(* Logix 5000 AddOnInstructionDefinition export SPEL_Above; software revision 30.01; part 5 of 9 *)

ADD_ON_INSTRUCTION SPEL_LocalSet   (* revision 1.0, vendor SEIKO EPSON CORP. *)
// Sets the local coordinate system of the specified coordinate number by each coordinate.
VAR_INPUT
   Start : BOOL; {required}
END_VAR
VAR_OUTPUT
   InCycle : BOOL; {access Read Only, visible}
   Done : BOOL; {access Read Only, visible}
   Error : BOOL; {access Read Only, visible}
END_VAR
VAR_INPUT
   NumAxes : INT; {required}
   LocalNum : INT; {required}
   LocalX : REAL; {required}
   LocalY : REAL; {required}
   LocalZ : REAL; {required}
   LocalU : REAL; {required}
   LocalV : REAL; {required}
   LocalW : REAL; {required}
END_VAR
VAR_IN_OUT
   ExtInputs : AB:ETHERNET_MODULE_INT_128Bytes:I:0; {required}
   ExtOutputs : AB:ETHERNET_MODULE_INT_128Bytes:O:0; {required}
END_VAR
VAR_OUTPUT
   ErrCode1 : INT; {access Read Only, visible}
   ErrCode2 : INT; {access Read Only, visible}
END_VAR
VAR
   Coordinatex1000 : DINT; {access None}
   Coordinate_INTS : INT[2]; {access None}
   ExecLocalSetZ : SPEL_ExecCmd := (MaxTime := 3000); {access None}
   ExecLocalSetY : SPEL_ExecCmd := (MaxTime := 3000); {access None}
   ExecLocalSetX : SPEL_ExecCmd := (MaxTime := 3000); {access None}
   X6 : BOOL; {access None}
   StartInit : BOOL[32]; {access None}
   OneShotStart : BOOL[32]; {access None}
   ExecLocalSetW : SPEL_ExecCmd := (MaxTime := 3000); {access None}
   ExecLocalSetV : SPEL_ExecCmd := (MaxTime := 3000); {access None}
   ExecLocalSetU : SPEL_ExecCmd := (MaxTime := 3000); {access None}
   ExecTimeout : DINT; {access None}
END_VAR

ROUTINE Logic   (* ladder *)
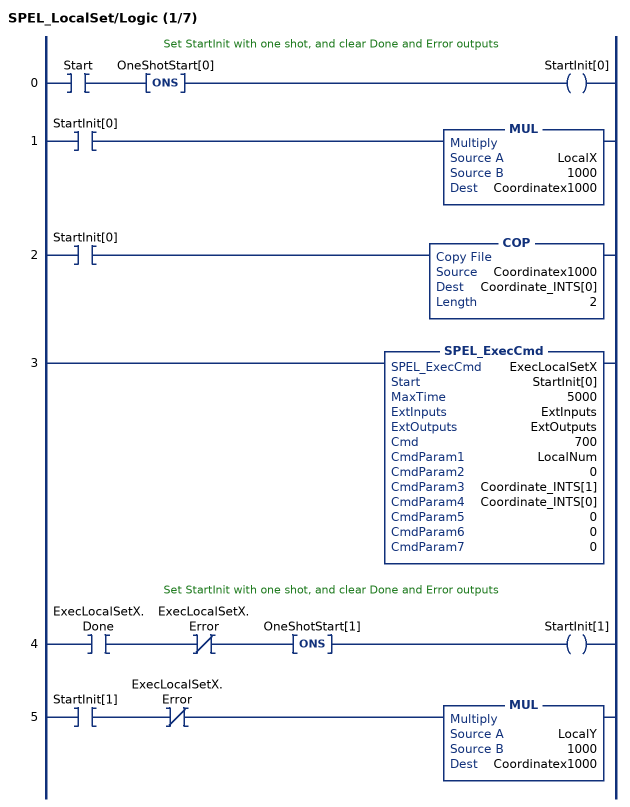
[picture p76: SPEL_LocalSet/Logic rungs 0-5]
   // Set StartInit with one shot, and clear Done and Error outputs
   0: XIC(Start)ONS(OneShotStart[0])OTE(StartInit[0]);
   1: XIC(StartInit[0])MUL(LocalX,1000,Coordinatex1000);
   2: XIC(StartInit[0])COP(Coordinatex1000,Coordinate_INTS[0],2);
   3: SPEL_ExecCmd(ExecLocalSetX,StartInit[0],5000,ExtInputs,ExtOutputs,700,LocalNum,0,Coordinate_INTS[1],Coordinate_INTS[0],0,0,0);
   // Set StartInit with one shot, and clear Done and Error outputs
   4: XIC(ExecLocalSetX.Done)XIO(ExecLocalSetX.Error)ONS(OneShotStart[1])OTE(StartInit[1]);
   5: XIC(StartInit[1])XIO(ExecLocalSetX.Error)MUL(LocalY,1000,Coordinatex1000);
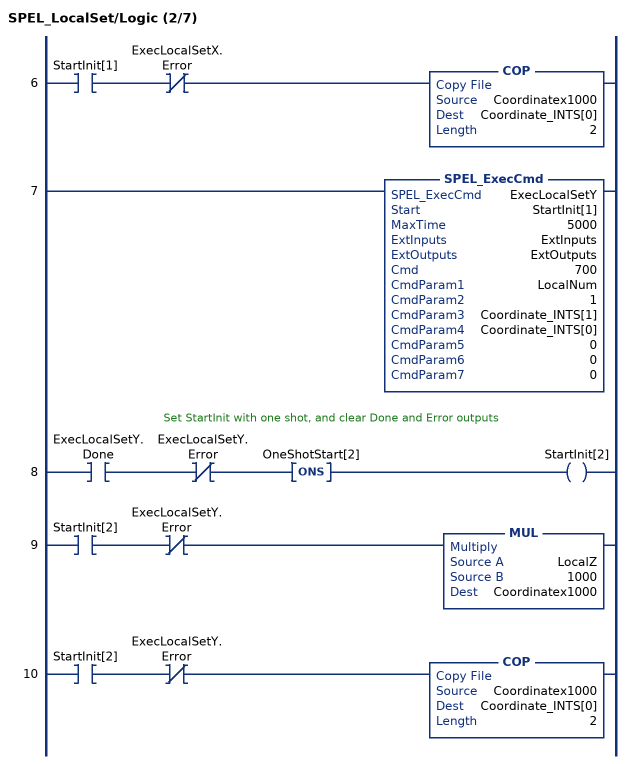
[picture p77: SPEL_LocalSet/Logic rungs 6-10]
   6: XIC(StartInit[1])XIO(ExecLocalSetX.Error)COP(Coordinatex1000,Coordinate_INTS[0],2);
   7: SPEL_ExecCmd(ExecLocalSetY,StartInit[1],5000,ExtInputs,ExtOutputs,700,LocalNum,1,Coordinate_INTS[1],Coordinate_INTS[0],0,0,0);
   // Set StartInit with one shot, and clear Done and Error outputs
   8: XIC(ExecLocalSetY.Done)XIO(ExecLocalSetY.Error)ONS(OneShotStart[2])OTE(StartInit[2]);
   9: XIC(StartInit[2])XIO(ExecLocalSetY.Error)MUL(LocalZ,1000,Coordinatex1000);
   10: XIC(StartInit[2])XIO(ExecLocalSetY.Error)COP(Coordinatex1000,Coordinate_INTS[0],2);
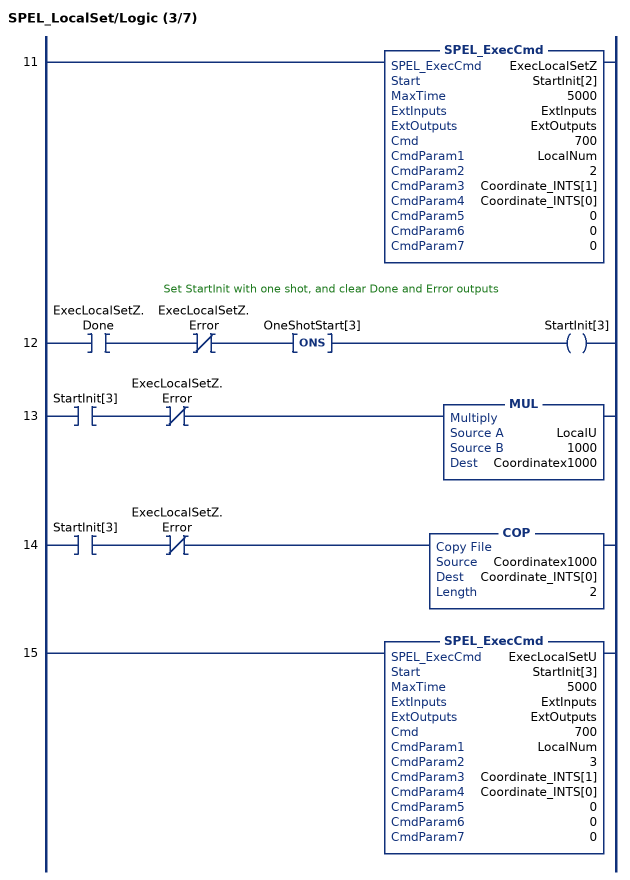
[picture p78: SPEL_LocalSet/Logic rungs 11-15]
   11: SPEL_ExecCmd(ExecLocalSetZ,StartInit[2],5000,ExtInputs,ExtOutputs,700,LocalNum,2,Coordinate_INTS[1],Coordinate_INTS[0],0,0,0);
   // Set StartInit with one shot, and clear Done and Error outputs
   12: XIC(ExecLocalSetZ.Done)XIO(ExecLocalSetZ.Error)ONS(OneShotStart[3])OTE(StartInit[3]);
   13: XIC(StartInit[3])XIO(ExecLocalSetZ.Error)MUL(LocalU,1000,Coordinatex1000);
   14: XIC(StartInit[3])XIO(ExecLocalSetZ.Error)COP(Coordinatex1000,Coordinate_INTS[0],2);
   15: SPEL_ExecCmd(ExecLocalSetU,StartInit[3],5000,ExtInputs,ExtOutputs,700,LocalNum,3,Coordinate_INTS[1],Coordinate_INTS[0],0,0,0);
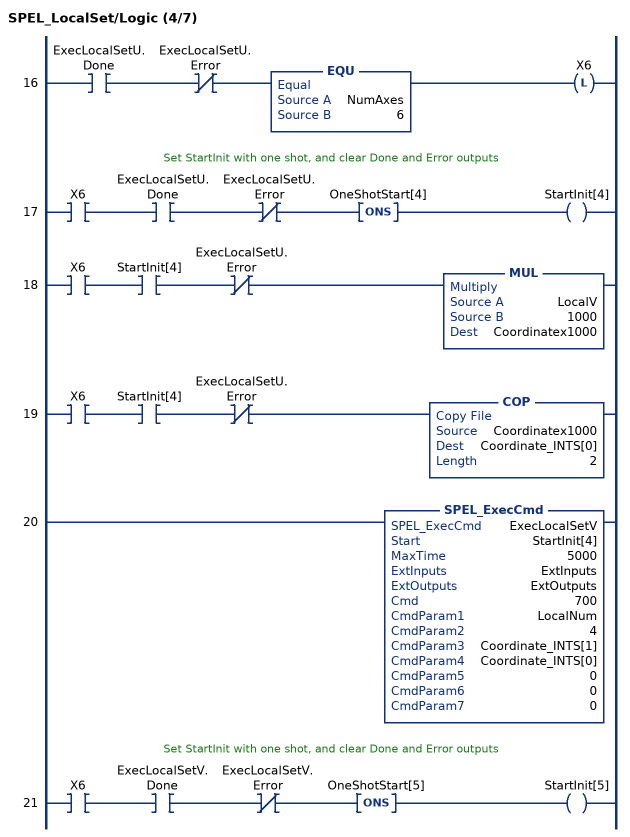
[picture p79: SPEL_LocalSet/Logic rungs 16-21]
   16: XIC(ExecLocalSetU.Done)XIO(ExecLocalSetU.Error)EQU(NumAxes,6)OTL(X6);
   // Set StartInit with one shot, and clear Done and Error outputs
   17: XIC(X6)XIC(ExecLocalSetU.Done)XIO(ExecLocalSetU.Error)ONS(OneShotStart[4])OTE(StartInit[4]);
   18: XIC(X6)XIC(StartInit[4])XIO(ExecLocalSetU.Error)MUL(LocalV,1000,Coordinatex1000);
   19: XIC(X6)XIC(StartInit[4])XIO(ExecLocalSetU.Error)COP(Coordinatex1000,Coordinate_INTS[0],2);
   20: SPEL_ExecCmd(ExecLocalSetV,StartInit[4],5000,ExtInputs,ExtOutputs,700,LocalNum,4,Coordinate_INTS[1],Coordinate_INTS[0],0,0,0);
   // Set StartInit with one shot, and clear Done and Error outputs
   21: XIC(X6)XIC(ExecLocalSetV.Done)XIO(ExecLocalSetV.Error)ONS(OneShotStart[5])OTE(StartInit[5]);
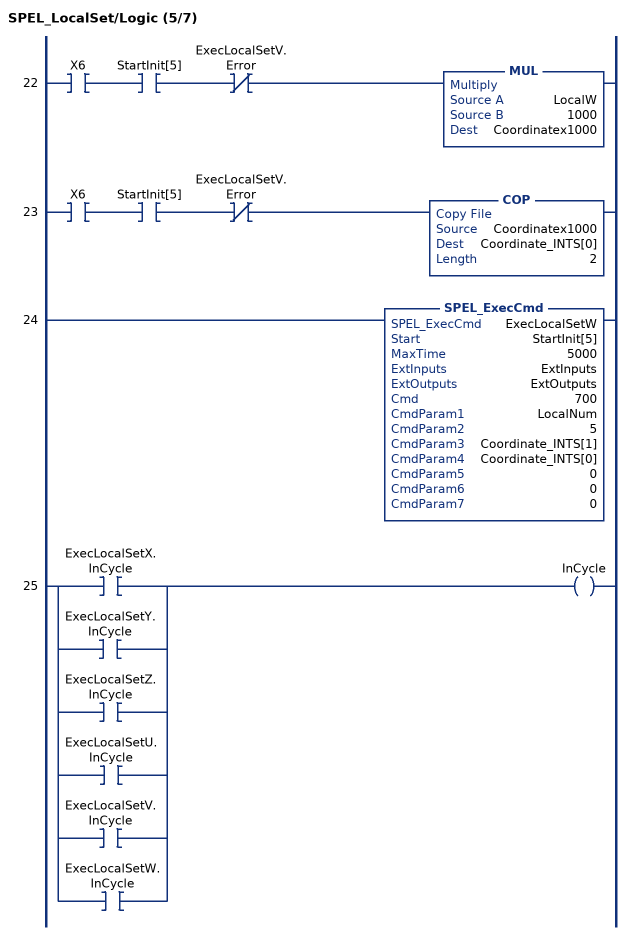
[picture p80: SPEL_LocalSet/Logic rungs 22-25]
   22: XIC(X6)XIC(StartInit[5])XIO(ExecLocalSetV.Error)MUL(LocalW,1000,Coordinatex1000);
   23: XIC(X6)XIC(StartInit[5])XIO(ExecLocalSetV.Error)COP(Coordinatex1000,Coordinate_INTS[0],2);
   24: SPEL_ExecCmd(ExecLocalSetW,StartInit[5],5000,ExtInputs,ExtOutputs,700,LocalNum,5,Coordinate_INTS[1],Coordinate_INTS[0],0,0,0);
   25: [XIC(ExecLocalSetX.InCycle) ,XIC(ExecLocalSetY.InCycle) ,XIC(ExecLocalSetZ.InCycle) ,XIC(ExecLocalSetU.InCycle) ,XIC(ExecLocalSetV.InCycle) ,XIC(ExecLocalSetW.InCycle) ]OTE(InCycle);
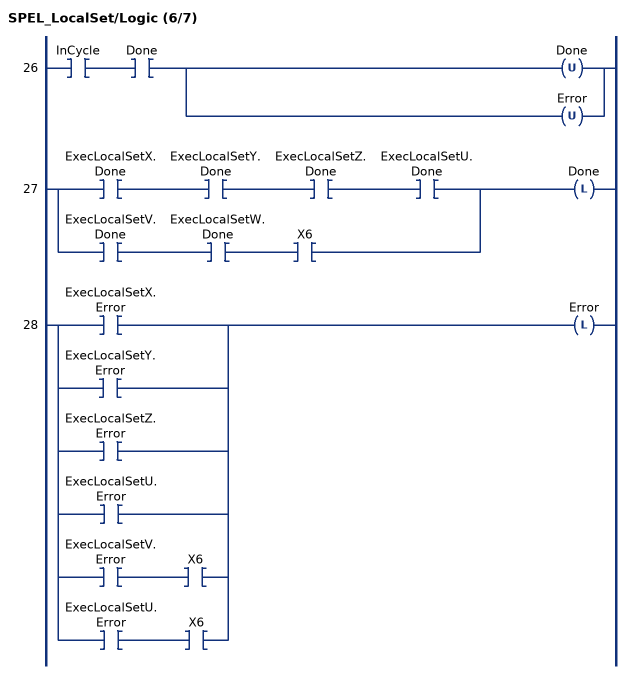
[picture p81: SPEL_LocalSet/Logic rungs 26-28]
   26: XIC(InCycle)XIC(Done)[OTU(Done) ,OTU(Error) ];
   27: [XIC(ExecLocalSetX.Done) XIC(ExecLocalSetY.Done) XIC(ExecLocalSetZ.Done) XIC(ExecLocalSetU.Done) ,XIC(ExecLocalSetV.Done) XIC(ExecLocalSetW.Done) XIC(X6) ]OTL(Done);
   28: [XIC(ExecLocalSetX.Error) ,XIC(ExecLocalSetY.Error) ,XIC(ExecLocalSetZ.Error) ,XIC(ExecLocalSetU.Error) ,XIC(ExecLocalSetV.Error) XIC(X6) ,XIC(ExecLocalSetU.Error) XIC(X6) ]OTL(Error);
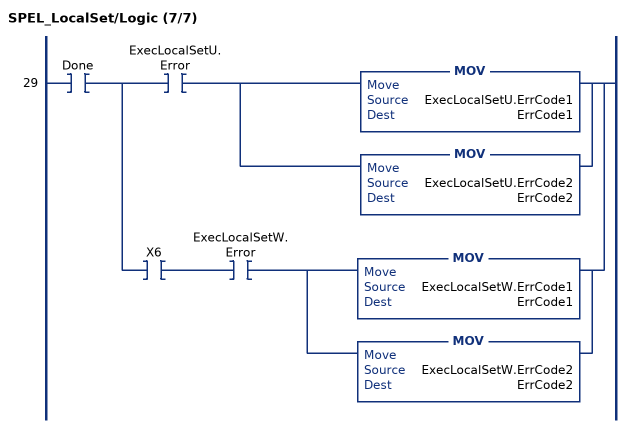
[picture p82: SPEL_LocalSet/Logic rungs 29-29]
   29: XIC(Done)[XIC(ExecLocalSetU.Error) [MOV(ExecLocalSetU.ErrCode1,ErrCode1) ,MOV(ExecLocalSetU.ErrCode2,ErrCode2) ] ,XIC(X6) XIC(ExecLocalSetW.Error) [MOV(ExecLocalSetW.ErrCode1,ErrCode1) ,MOV(ExecLocalSetW.ErrCode2,ErrCode2) ] ];
END_ROUTINE
END_ADD_ON_INSTRUCTION

ADD_ON_INSTRUCTION SPEL_MemIn   (* revision 1.0, vendor SEIKO EPSON CORP. *)
// Reads a byte of memory IO.
VAR_OUTPUT
   InCycle : BOOL; {access Read Only, visible}
   Done : BOOL; {access Read Only, visible}
   Error : BOOL; {access Read Only, visible}
END_VAR
VAR_INPUT
   Start : BOOL; {access Read Only, required}
   PortNum : INT; {required}
END_VAR
VAR_OUTPUT
   Value : INT; {access Read Only, visible}
END_VAR
VAR_IN_OUT
   ExtInputs : AB:ETHERNET_MODULE_INT_128Bytes:I:0; {required}
   ExtOutputs : AB:ETHERNET_MODULE_INT_128Bytes:O:0; {required}
END_VAR
VAR_OUTPUT
   ErrCode1 : INT; {access Read Only, visible}
   ErrCode2 : INT; {access Read Only, visible}
END_VAR
VAR
   ExecMemIn : SPEL_ExecCmd := (MaxTime := 3000); {access None}
        .INCYCLE   // ExecInCycle
        .DONE   // ExecDone
        .ERROR   // ExecError
   OneShotStart : BOOL; {access None}
   StartCoil : BOOL; {access None}
   ExecTimeout : DINT; {access None}
END_VAR

ROUTINE Logic   (* ladder *)
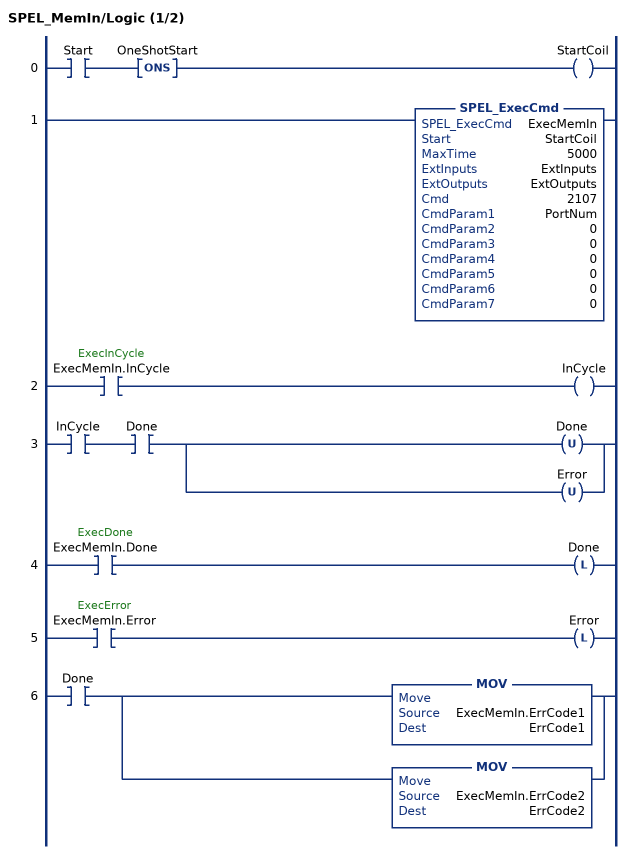
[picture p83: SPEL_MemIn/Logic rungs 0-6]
   0: XIC(Start)ONS(OneShotStart)OTE(StartCoil);
   1: SPEL_ExecCmd(ExecMemIn,StartCoil,5000,ExtInputs,ExtOutputs,2107,PortNum,0,0,0,0,0,0);
   2: XIC(ExecMemIn.InCycle)OTE(InCycle);
   3: XIC(InCycle)XIC(Done)[OTU(Done) ,OTU(Error) ];
   4: XIC(ExecMemIn.Done)OTL(Done);
   5: XIC(ExecMemIn.Error)OTL(Error);
   6: XIC(Done)[MOV(ExecMemIn.ErrCode1,ErrCode1) ,MOV(ExecMemIn.ErrCode2,ErrCode2) ];
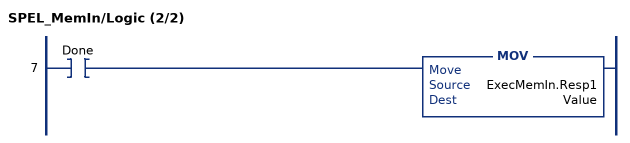
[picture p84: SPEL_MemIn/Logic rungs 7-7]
   7: XIC(Done)MOV(ExecMemIn.Resp1,Value);
END_ROUTINE
END_ADD_ON_INSTRUCTION

ADD_ON_INSTRUCTION SPEL_MemInW   (* revision 1.0, vendor SEIKO EPSON CORP. *)
// Reads a word of memory IO.
VAR_OUTPUT
   InCycle : BOOL; {access Read Only, visible}
   Done : BOOL; {access Read Only, visible}
   Error : BOOL; {access Read Only, visible}
END_VAR
VAR_INPUT
   Start : BOOL; {access Read Only, required}
   PortNum : INT; {required}
END_VAR
VAR_OUTPUT
   Value : DINT; {access Read Only, visible}
END_VAR
VAR_IN_OUT
   ExtInputs : AB:ETHERNET_MODULE_INT_128Bytes:I:0; {required}
   ExtOutputs : AB:ETHERNET_MODULE_INT_128Bytes:O:0; {required}
END_VAR
VAR_OUTPUT
   ErrCode1 : INT; {access Read Only, visible}
   ErrCode2 : INT; {access Read Only, visible}
END_VAR
VAR
   ExecMemInW : SPEL_ExecCmd := (MaxTime := 3000); {access None}
        .INCYCLE   // ExecInCycle
        .DONE   // ExecDone
        .ERROR   // ExecError
   OneShotStart : BOOL; {access None}
   StartCoil : BOOL; {access None}
   ExecTimeout : DINT; {access None}
END_VAR

ROUTINE Logic   (* ladder *)
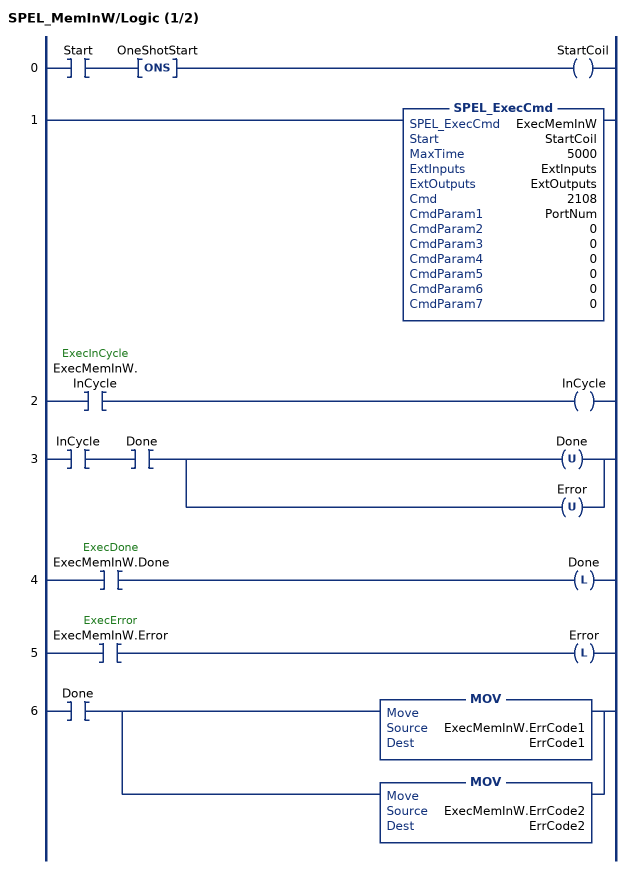
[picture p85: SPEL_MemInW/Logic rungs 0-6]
   0: XIC(Start)ONS(OneShotStart)OTE(StartCoil);
   1: SPEL_ExecCmd(ExecMemInW,StartCoil,5000,ExtInputs,ExtOutputs,2108,PortNum,0,0,0,0,0,0);
   2: XIC(ExecMemInW.InCycle)OTE(InCycle);
   3: XIC(InCycle)XIC(Done)[OTU(Done) ,OTU(Error) ];
   4: XIC(ExecMemInW.Done)OTL(Done);
   5: XIC(ExecMemInW.Error)OTL(Error);
   6: XIC(Done)[MOV(ExecMemInW.ErrCode1,ErrCode1) ,MOV(ExecMemInW.ErrCode2,ErrCode2) ];
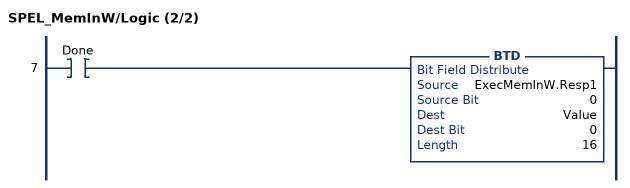
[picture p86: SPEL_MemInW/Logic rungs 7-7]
   7: XIC(Done)BTD(ExecMemInW.Resp1,0,Value,0,16);
END_ROUTINE
END_ADD_ON_INSTRUCTION

ADD_ON_INSTRUCTION SPEL_MemOff   (* revision 1.0, vendor SEIKO EPSON CORP. *)
// Turns a memory IO bit off.
VAR_OUTPUT
   InCycle : BOOL; {access Read Only, visible}
   Done : BOOL; {access Read Only, visible}
   Error : BOOL; {access Read Only, visible}
END_VAR
VAR_INPUT
   Start : BOOL; {access Read Only, required}
   BitNum : INT; {required}
END_VAR
VAR_IN_OUT
   ExtInputs : AB:ETHERNET_MODULE_INT_128Bytes:I:0; {required}
   ExtOutputs : AB:ETHERNET_MODULE_INT_128Bytes:O:0; {required}
END_VAR
VAR_OUTPUT
   ErrCode1 : INT; {access Read Only, visible}
   ErrCode2 : INT; {access Read Only, visible}
END_VAR
VAR
   ExecMemOff : SPEL_ExecCmd := (MaxTime := 3000); {access None}
        .INCYCLE   // ExecInCycle
        .DONE   // ExecDone
        .ERROR   // ExecError
   OneShotStart : BOOL; {access None}
   StartCoil : BOOL; {access None}
   ExecTimeout : DINT; {access None}
END_VAR

ROUTINE Logic   (* ladder *)
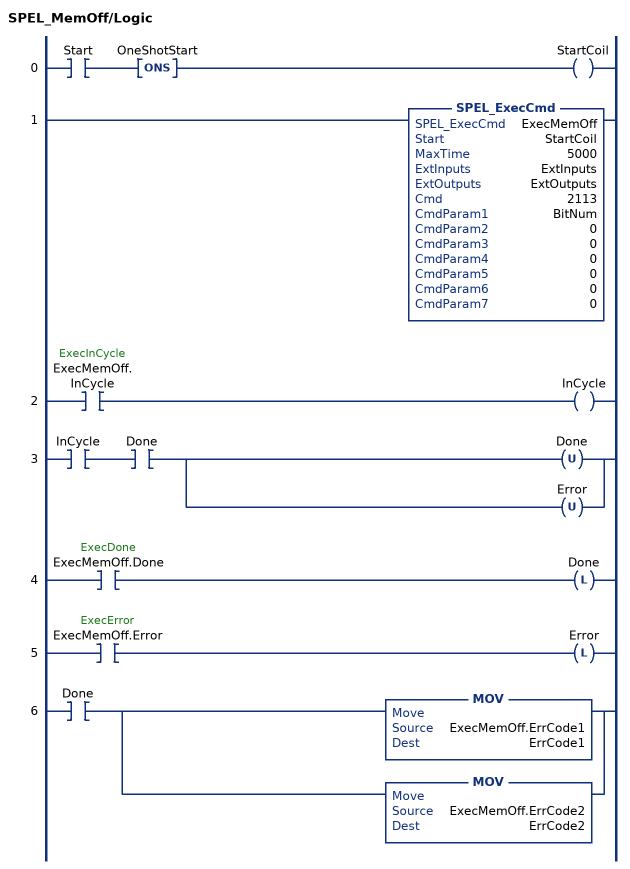
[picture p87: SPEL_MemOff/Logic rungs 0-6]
   0: XIC(Start)ONS(OneShotStart)OTE(StartCoil);
   1: SPEL_ExecCmd(ExecMemOff,StartCoil,5000,ExtInputs,ExtOutputs,2113,BitNum,0,0,0,0,0,0);
   2: XIC(ExecMemOff.InCycle)OTE(InCycle);
   3: XIC(InCycle)XIC(Done)[OTU(Done) ,OTU(Error) ];
   4: XIC(ExecMemOff.Done)OTL(Done);
   5: XIC(ExecMemOff.Error)OTL(Error);
   6: XIC(Done)[MOV(ExecMemOff.ErrCode1,ErrCode1) ,MOV(ExecMemOff.ErrCode2,ErrCode2) ];
END_ROUTINE
END_ADD_ON_INSTRUCTION

ADD_ON_INSTRUCTION SPEL_MemOn   (* revision 1.0, vendor SEIKO EPSON CORP. *)
// Turns a memory IO bit on.
VAR_OUTPUT
   InCycle : BOOL; {access Read Only, visible}
   Done : BOOL; {access Read Only, visible}
   Error : BOOL; {access Read Only, visible}
END_VAR
VAR_INPUT
   Start : BOOL; {access Read Only, required}
   BitNum : INT; {required}
END_VAR
VAR_IN_OUT
   ExtInputs : AB:ETHERNET_MODULE_INT_128Bytes:I:0; {required}
   ExtOutputs : AB:ETHERNET_MODULE_INT_128Bytes:O:0; {required}
END_VAR
VAR_OUTPUT
   ErrCode1 : INT; {access Read Only, visible}
   ErrCode2 : INT; {access Read Only, visible}
END_VAR
VAR
   ExecMemOn : SPEL_ExecCmd := (MaxTime := 3000); {access None}
        .INCYCLE   // ExecInCycle
        .DONE   // ExecDone
        .ERROR   // ExecError
   OneShotStart : BOOL; {access None}
   ExecTimeout : DINT; {access None}
   StartCoil : BOOL; {access None}
END_VAR

ROUTINE Logic   (* ladder *)
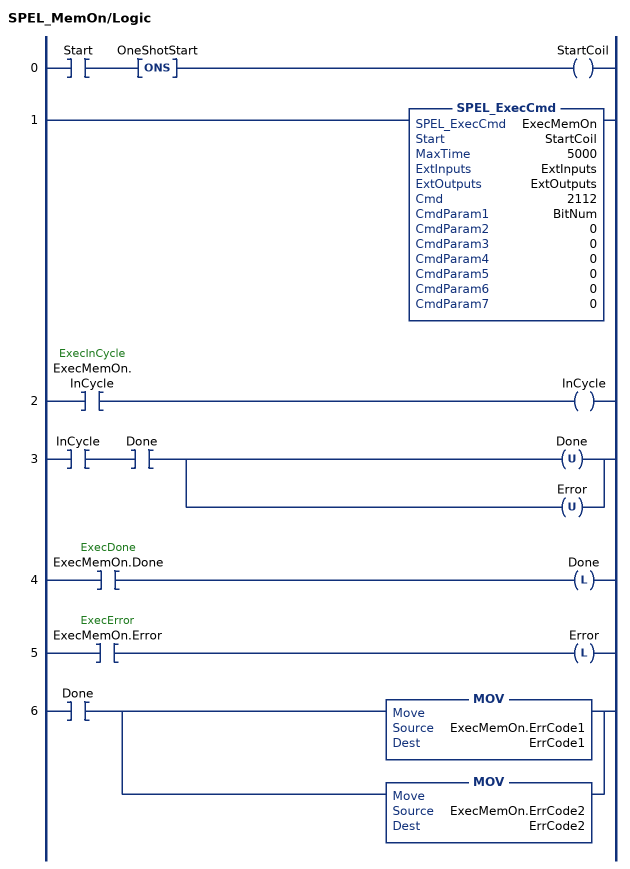
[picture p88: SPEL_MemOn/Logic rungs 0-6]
   0: XIC(Start)ONS(OneShotStart)OTE(StartCoil);
   1: SPEL_ExecCmd(ExecMemOn,StartCoil,5000,ExtInputs,ExtOutputs,2112,BitNum,0,0,0,0,0,0);
   2: XIC(ExecMemOn.InCycle)OTE(InCycle);
   3: XIC(InCycle)XIC(Done)[OTU(Done) ,OTU(Error) ];
   4: XIC(ExecMemOn.Done)OTL(Done);
   5: XIC(ExecMemOn.Error)OTL(Error);
   6: XIC(Done)[MOV(ExecMemOn.ErrCode1,ErrCode1) ,MOV(ExecMemOn.ErrCode2,ErrCode2) ];
END_ROUTINE
END_ADD_ON_INSTRUCTION

ADD_ON_INSTRUCTION SPEL_MemOut   (* revision 1.0, vendor SEIKO EPSON CORP. *)
// Sets a byte of memory IO.
VAR_OUTPUT
   InCycle : BOOL; {access Read Only, visible}
   Done : BOOL; {access Read Only, visible}
   Error : BOOL; {access Read Only, visible}
END_VAR
VAR_INPUT
   Start : BOOL; {access Read Only, required}
   PortNum : INT; {required}
   OutData : INT; {required}
END_VAR
VAR_IN_OUT
   ExtInputs : AB:ETHERNET_MODULE_INT_128Bytes:I:0; {required}
   ExtOutputs : AB:ETHERNET_MODULE_INT_128Bytes:O:0; {required}
END_VAR
VAR_OUTPUT
   ErrCode1 : INT; {access Read Only, visible}
   ErrCode2 : INT; {access Read Only, visible}
END_VAR
VAR
   ExecMemOut : SPEL_ExecCmd := (MaxTime := 3000); {access None}
        .INCYCLE   // ExecInCycle
        .DONE   // ExecDone
        .ERROR   // ExecError
   OneShotStart : BOOL; {access None}
   StartCoil : BOOL; {access None}
   ExecTimeout : DINT; {access None}
END_VAR

ROUTINE Logic   (* ladder *)
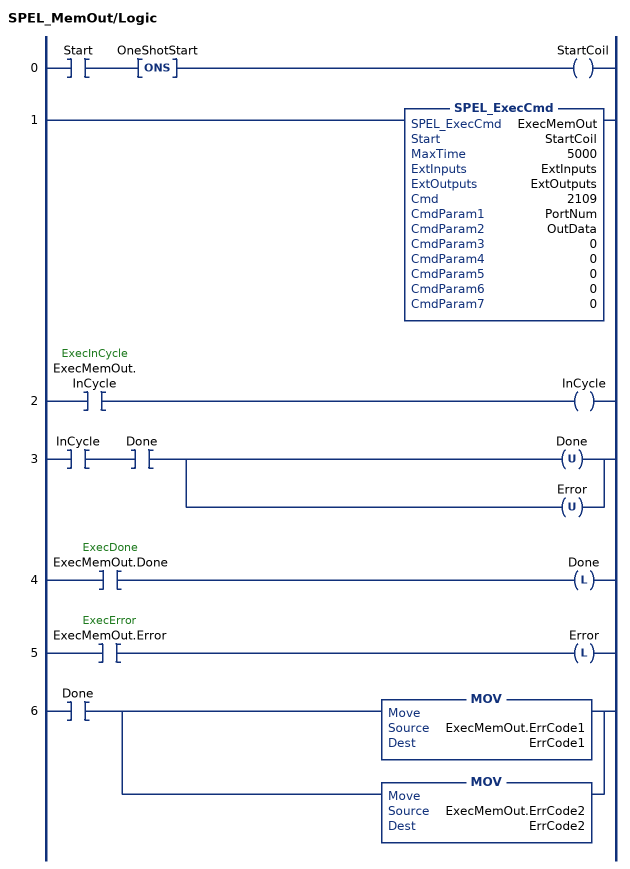
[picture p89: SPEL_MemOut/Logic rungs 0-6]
   0: XIC(Start)ONS(OneShotStart)OTE(StartCoil);
   1: SPEL_ExecCmd(ExecMemOut,StartCoil,5000,ExtInputs,ExtOutputs,2109,PortNum,OutData,0,0,0,0,0);
   2: XIC(ExecMemOut.InCycle)OTE(InCycle);
   3: XIC(InCycle)XIC(Done)[OTU(Done) ,OTU(Error) ];
   4: XIC(ExecMemOut.Done)OTL(Done);
   5: XIC(ExecMemOut.Error)OTL(Error);
   6: XIC(Done)[MOV(ExecMemOut.ErrCode1,ErrCode1) ,MOV(ExecMemOut.ErrCode2,ErrCode2) ];
END_ROUTINE
END_ADD_ON_INSTRUCTION

ADD_ON_INSTRUCTION SPEL_MemOutW   (* revision 1.0, vendor SEIKO EPSON CORP. *)
// Sets a word of memory IO.
VAR_OUTPUT
   InCycle : BOOL; {access Read Only, visible}
   Done : BOOL; {access Read Only, visible}
   Error : BOOL; {access Read Only, visible}
END_VAR
VAR_INPUT
   Start : BOOL; {access Read Only, required}
   PortNum : INT; {required}
   OutData : INT; {required}
END_VAR
VAR_IN_OUT
   ExtInputs : AB:ETHERNET_MODULE_INT_128Bytes:I:0; {required}
   ExtOutputs : AB:ETHERNET_MODULE_INT_128Bytes:O:0; {required}
END_VAR
VAR_OUTPUT
   ErrCode1 : INT; {access Read Only, visible}
   ErrCode2 : INT; {access Read Only, visible}
END_VAR
VAR
   ExecMemOutW : SPEL_ExecCmd := (MaxTime := 3000); {access None}
        .INCYCLE   // ExecInCycle
        .DONE   // ExecDone
        .ERROR   // ExecError
   OneShotStart : BOOL; {access None}
   StartCoil : BOOL; {access None}
   ExecTimeout : DINT; {access None}
END_VAR

ROUTINE Logic   (* ladder *)
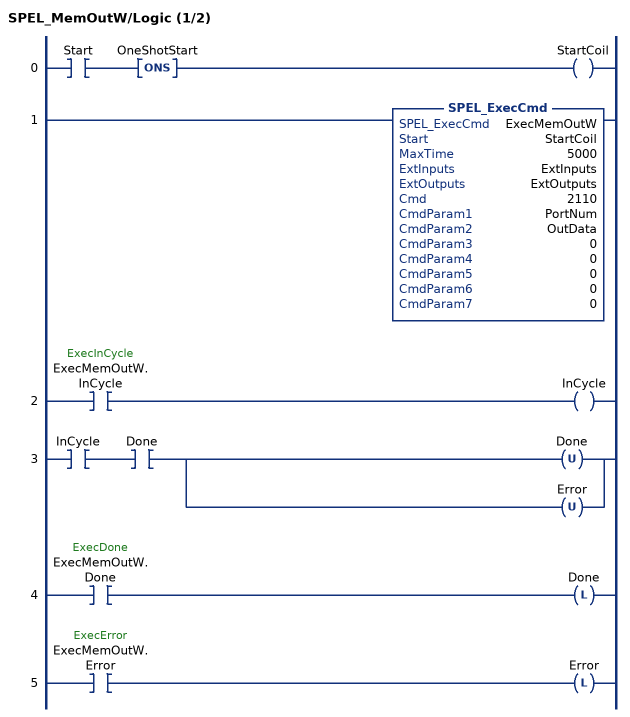
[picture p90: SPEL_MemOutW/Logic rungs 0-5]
   0: XIC(Start)ONS(OneShotStart)OTE(StartCoil);
   1: SPEL_ExecCmd(ExecMemOutW,StartCoil,5000,ExtInputs,ExtOutputs,2110,PortNum,OutData,0,0,0,0,0);
   2: XIC(ExecMemOutW.InCycle)OTE(InCycle);
   3: XIC(InCycle)XIC(Done)[OTU(Done) ,OTU(Error) ];
   4: XIC(ExecMemOutW.Done)OTL(Done);
   5: XIC(ExecMemOutW.Error)OTL(Error);
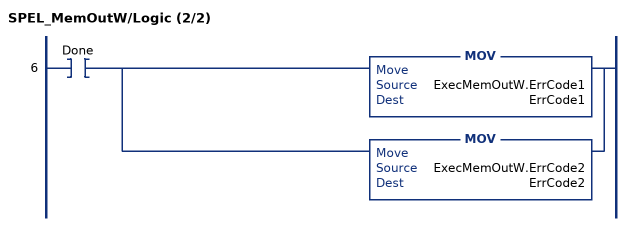
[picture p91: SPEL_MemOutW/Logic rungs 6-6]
   6: XIC(Done)[MOV(ExecMemOutW.ErrCode1,ErrCode1) ,MOV(ExecMemOutW.ErrCode2,ErrCode2) ];
END_ROUTINE
END_ADD_ON_INSTRUCTION

ADD_ON_INSTRUCTION SPEL_MemSw   (* revision 1.0, vendor SEIKO EPSON CORP. *)
// Reads bit of memory IO.
VAR_OUTPUT
   InCycle : BOOL; {access Read Only, visible}
   Done : BOOL; {access Read Only, visible}
   Error : BOOL; {access Read Only, visible}
END_VAR
VAR_INPUT
   Start : BOOL; {access Read Only, required}
   Bit : INT; {required}
END_VAR
VAR_OUTPUT
   Value : INT; {access Read Only, visible}
END_VAR
VAR_IN_OUT
   ExtInputs : AB:ETHERNET_MODULE_INT_128Bytes:I:0; {required}
   ExtOutputs : AB:ETHERNET_MODULE_INT_128Bytes:O:0; {required}
END_VAR
VAR_OUTPUT
   ErrCode1 : INT; {access Read Only, visible}
   ErrCode2 : INT; {access Read Only, visible}
END_VAR
VAR
   ExecMemSw : SPEL_ExecCmd := (MaxTime := 3000); {access None}
        .INCYCLE   // ExecInCycle
        .DONE   // ExecDone
        .ERROR   // ExecError
   OneShotStart : BOOL; {access None}
   StartCoil : BOOL; {access None}
   ExecTimeout : DINT; {access None}
END_VAR

ROUTINE Logic   (* ladder *)
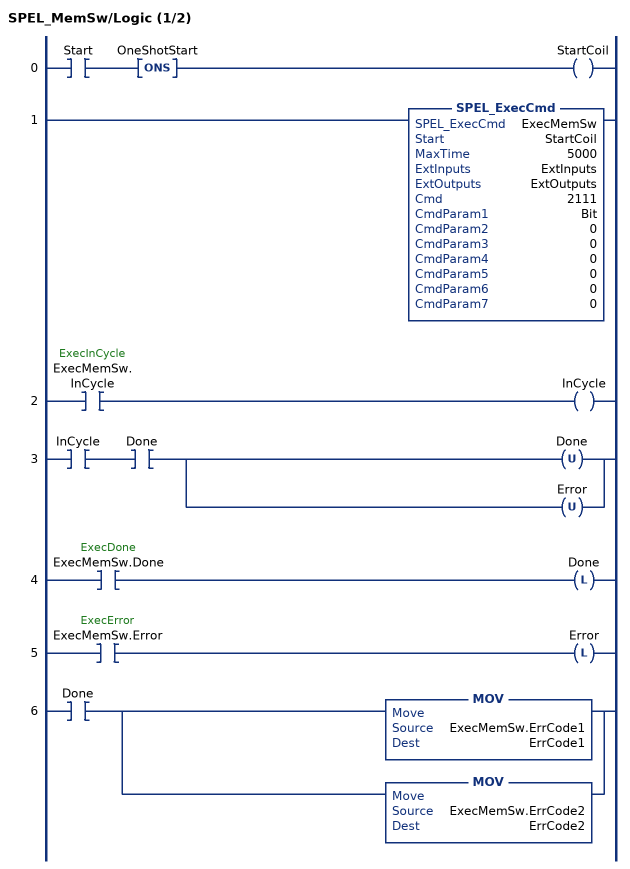
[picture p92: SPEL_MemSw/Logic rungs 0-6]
   0: XIC(Start)ONS(OneShotStart)OTE(StartCoil);
   1: SPEL_ExecCmd(ExecMemSw,StartCoil,5000,ExtInputs,ExtOutputs,2111,Bit,0,0,0,0,0,0);
   2: XIC(ExecMemSw.InCycle)OTE(InCycle);
   3: XIC(InCycle)XIC(Done)[OTU(Done) ,OTU(Error) ];
   4: XIC(ExecMemSw.Done)OTL(Done);
   5: XIC(ExecMemSw.Error)OTL(Error);
   6: XIC(Done)[MOV(ExecMemSw.ErrCode1,ErrCode1) ,MOV(ExecMemSw.ErrCode2,ErrCode2) ];
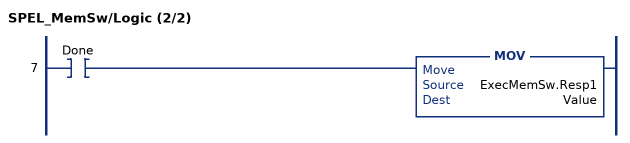
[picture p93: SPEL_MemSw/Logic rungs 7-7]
   7: XIC(Done)MOV(ExecMemSw.Resp1,Value);
END_ROUTINE
END_ADD_ON_INSTRUCTION
